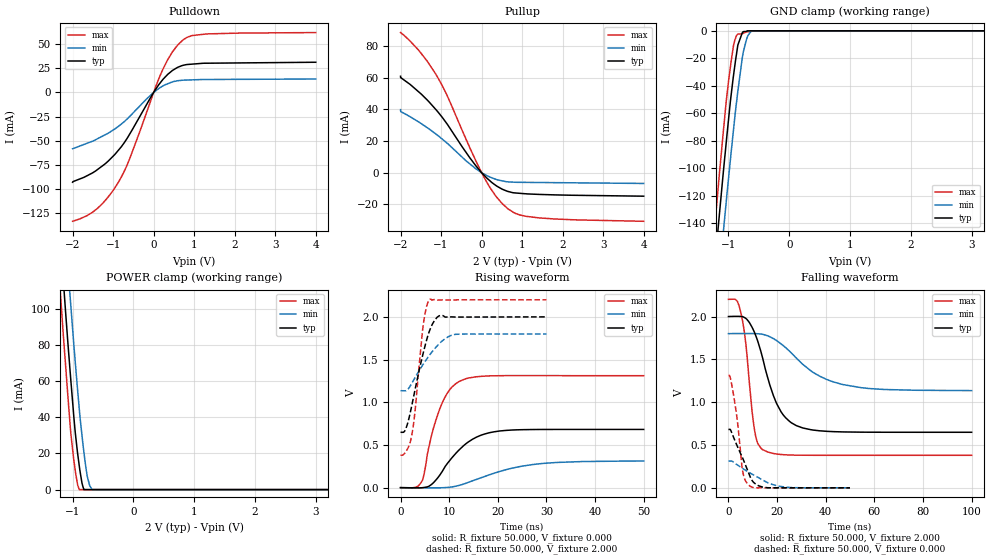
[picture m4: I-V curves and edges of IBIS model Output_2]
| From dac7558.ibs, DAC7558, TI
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|   TRISTATE OUTPUT 2.0V Model
[Model]   Output_2
Model_type   3-state
Polarity   Non-Inverting
Enable   Active-High
Vmeas = 1
Vref = 1
Cref = 15pF
Rref = 50
|   typ   min   max
|   (nom PVT)   (fast PVT)  (slow PVT)
|Average
C_comp   4.991e-12   4.329e-12   6.341e-12
|ON state : BUFFER OUTPUT TURNED HIGH
|C_comp   8.792e-12   7.481e-12   1.147e-11
|OFF state: BUFFER in HIGH IMPEDANCE for IOs and 3-state,
|This is BUFFER in LOW state for OUTPUT only type
|C_comp   1.190e-12   1.176e-12   1.211e-12
|Where nom PVT is Nominal Process, 2V, 25C
|   fast PVT is Strong Process, 2.2V, -40C
|   slow PVT is Weak Process, 1.8V, 105C
[Voltage Range]   2   1.8   2.2
|Ambient Temperature   25   105   -40
|Junction Temperature
[Temperature Range]   25   105   -40
[Pullup Reference]   2   1.8   2.2
[Pulldown Reference]   0   0   0
[Power Clamp Reference]   2   1.8   2.2
[GND Clamp Reference]   0   0   0
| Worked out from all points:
|   slope of the pulldown table from 0 to 0.3 V, typ, clamps not added: 18 ohm
|   slope of the pullup table from 0 to 0.3 V, typ, clamps not added: 42.2 ohm
|   GND clamp passes 1 mA (typ) near -0.76 V on its own axis
|   POWER clamp passes 1 mA (typ) near -0.82 V on its own axis
|   falling waveform, R_fixture 50.000, V_fixture 2.000: 20-80 % time 9.2ns typ, 18ns min, 3.92ns max; typ from 2 V to 0.649 V
|   rising waveform, R_fixture 50.000, V_fixture 0.000: 20-80 % time 6.28ns typ, 10.9ns min, 3.87ns max; typ from 0 V to 0.682 V
|   rising waveform, R_fixture 50.000, V_fixture 2.000: 20-80 % time 3.21ns typ, 4.87ns min, 1.85ns max; typ from 0.649 V to 2 V
|   falling waveform, R_fixture 50.000, V_fixture 0.000: 20-80 % time 6.08ns typ, 11.4ns min, 3.2ns max; typ from 0.682 V to 0 V
[Pulldown]
|   Voltage   I(typ)   I(min)   I(max)
-2V       -93.09mA   -58.43mA   -133.6mA
-1.397V   -80.3mA    -48.26mA   -120.6mA
-1.135V   -71.71mA   -42.56mA   -109.1mA
-889mV    -60.89mA   -35.81mA   -94.42mA
-598.6mV  -43.68mA   -25.22mA   -69.48mA
0V        0A         0A         0A
217.6mV   12.93mA    6.507mA    23.1mA
468.4mV   22.9mA     11.01mA    42.35mA
723.6mV   28.07mA    12.71mA    54.39mA
943.6mV   29.32mA    13.02mA    58.91mA
1.307V    30.29mA    13.42mA    60.65mA
4V        31.29mA    13.91mA    62.06mA
[GND Clamp]
|   Voltage   I(typ)   I(min)   I(max)
-2V       -570.3mA   -601.6mA   -556.5mA
-1.23V    -172.8mA   -215.2mA   -144.7mA
-1.174V   -145.5mA   -188.3mA   -116.6mA
-1.155V   -136.5mA   -179.4mA   -107.2mA
-1.086V   -103.6mA   -147.1mA   -74.15mA
-1.036V   -81.12mA   -124.2mA   -51.24mA
-955mV    -46.41mA   -88.1mA    -21.96mA
-913.2mV  -31.31mA   -70.38mA   -9.98mA
-844mV    -10.17mA   -43.52mA   -2.327mA
-756mV    -594.4uA   -15.45mA   -1.819mA
-619.4mV  0A         0A         -290.1uA
4V        0A         0A         0A
[Pullup]
|   Voltage   I(typ)   I(min)   I(max)
-2V       60.77mA    39.72mA    88.35mA
-1.993V   59.9mA     38.44mA    88.21mA
-1.551V   50.94mA    31.96mA    77.18mA
-1.138V   40.07mA    24.56mA    62.44mA
-867mV    31.28mA    18.92mA    49.57mA
-298mV    9.645mA    5.686mA    16.16mA
54.8mV    -1.466mA   -824.9uA   -2.696mA
351.8mV   -8.092mA   -4.201mA   -14.82mA
648.8mV   -11.85mA   -5.829mA   -22.78mA
941.4mV   -13.04mA   -6.112mA   -26.68mA
1.41V     -13.73mA   -6.221mA   -28.53mA
4V        -14.86mA   -6.824mA   -30.7mA
[POWER Clamp]
|   Voltage   I(typ)   I(min)   I(max)
-2V       543mA      574.7mA    525.4mA
-1.194V   134.9mA    176.2mA    105.3mA
-1.141V   110.3mA    151.6mA    80.29mA
-1.114V   97.57mA    139.2mA    68.02mA
-1.036V   63.45mA    104.7mA    33.8mA
-950.6mV  29.79mA    68.11mA    9.144mA
-889mV    12.78mA    44.1mA     0A
-830mV    1.594mA    25.03mA    0A
-779.6mV  0A         11.72mA    0A
-722mV    0A         2.556mA    0A
-678.8mV  0A         39.61uA    0A
4V        0A         0A         0A
[Ramp]
R_load = 50
|   typ   min   max
dV/dt_r   0.409141/6.26467e-09   0.190266/1.08469e-08   0.786884/3.86589e-09
dV/dt_f   0.810886/9.13743e-09   0.398738/1.78951e-08   1.09212/3.90363e-09
[Falling Waveform]
R_fixture = 50.000
V_fixture = 2.000
V_fixture_min = 1.800
V_fixture_max = 2.200
C_fixture = 0.000
|  time   V(typ)   V(min)   V(max)
0s        2V         1.8V       2.2V
3.35ns    2.002V     1.801V     2.188V
5.25ns    2.001V     1.801V     2.028V
7.125ns   1.978V     1.801V     1.687V
10.7ns    1.815V     1.801V     679.8mV
13.98ns   1.524V     1.792V     446.8mV
21.63ns   887.9mV    1.681V     389mV
30.58ns   698.9mV    1.441V     380.6mV
54.63ns   649.9mV    1.169V     379.8mV
99.98ns   648.5mV    1.135V     379.8mV
[Rising Waveform]
R_fixture = 50.000
V_fixture = 0.000
V_fixture_min = 0.000
V_fixture_max = 0.000
C_fixture = 0.000
|  time   V(typ)   V(min)   V(max)
0s        605.9pV    0V         422.8pV
4.4ns     -999uV     -1.603mV   76.19mV
6.35ns    36.49mV    -1.822mV   604.2mV
8ns       141mV      -1.693mV   911.2mV
10.18ns   322.1mV    5.002mV    1.152V
12.1ns    445mV      27.26mV    1.245V
15.63ns   591.7mV    96.73mV    1.299V
20.38ns   663.5mV    189.2mV    1.311V
29.4ns    681.5mV    284mV      1.312V
50ns      681.9mV    312mV      1.311V
[Rising Waveform]
R_fixture = 50.000
V_fixture = 2.000
V_fixture_min = 1.800
V_fixture_max = 2.200
C_fixture = 0.000
|  time   V(typ)   V(min)   V(max)
0s        648.5mV    1.135V     379.8mV
1.075ns   688.2mV    1.135V     419.7mV
2.325ns   965.3mV    1.223V     618.5mV
3ns       1.151V     1.29V      904.1mV
4.65ns    1.572V     1.444V     1.896V
5.2ns     1.694V     1.491V     2.083V
5.9ns     1.827V     1.547V     2.198V
7.875ns   2.01V      1.681V     2.197V
11.33ns   1.998V     1.796V     2.199V
30ns      2V         1.8V       2.2V
[Falling Waveform]
R_fixture = 50.000
V_fixture = 0.000
V_fixture_min = 0.000
V_fixture_max = 0.000
C_fixture = 0.000
|  time   V(typ)   V(min)   V(max)
0s        681.9mV    312mV      1.311V
950ps     671.5mV    312.3mV    1.261V
2.85ns    538.9mV    284.2mV    949.4mV
3.825ns   474.1mV    264.7mV    743.2mV
5.875ns   344.7mV    225.7mV    191.6mV
8.125ns   186.7mV    186mV      37.94mV
10.4ns    62.26mV    149.1mV    2.403mV
14.18ns   8.115mV    89.05mV    464.6uV
23.38ns   327uV      8.765mV    28.19uV
49.98ns   1.16nV     0V         422.6pV
